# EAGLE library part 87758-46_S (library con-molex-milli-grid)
HEADER
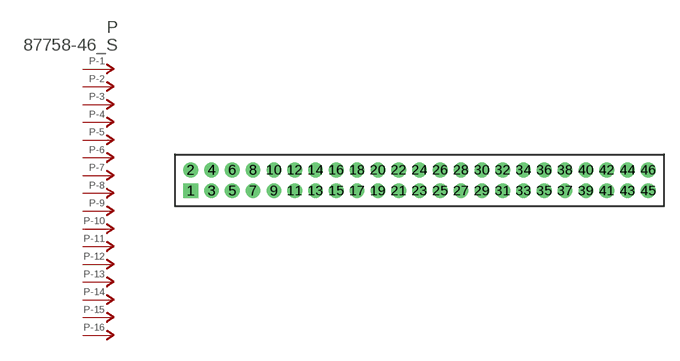
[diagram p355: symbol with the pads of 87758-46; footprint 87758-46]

Designator prefix P; gates -1=P-NV -2=P-N -3=P-N -4=P-N -5=P-N -6=P-N -7=P-N -8=P-N -9=P-N -10=P-N -11=P-N -12=P-N -13=P-N -14=P-N -15=P-N -16=P-N -17=P-N -18=P-N -19=P-N -20=P-N -21=P-N -22=P-N -23=P-N -24=P-N -25=P-N -26=P-N -27=P-N -28=P-N -29=P-N -30=P-N -31=P-N -32=P-N -33=P-N -34=P-N -35=P-N -36=P-N -37=P-N -38=P-N -39=P-N -40=P-N -41=P-N -42=P-N -43=P-N -44=P-N -45=P-N -46=P-N

## 87758-46_S  [87758-46]
1  -1:P  pas
2  -2:P  pas
3  -3:P  pas
4  -4:P  pas
5  -5:P  pas
6  -6:P  pas
7  -7:P  pas
8  -8:P  pas
9  -9:P  pas
10  -10:P  pas
11  -11:P  pas
12  -12:P  pas
13  -13:P  pas
14  -14:P  pas
15  -15:P  pas
16  -16:P  pas
17  -17:P  pas
18  -18:P  pas
19  -19:P  pas
20  -20:P  pas
21  -21:P  pas
22  -22:P  pas
23  -23:P  pas
24  -24:P  pas
25  -25:P  pas
26  -26:P  pas
27  -27:P  pas
28  -28:P  pas
29  -29:P  pas
30  -30:P  pas
31  -31:P  pas
32  -32:P  pas
33  -33:P  pas
34  -34:P  pas
35  -35:P  pas
36  -36:P  pas
37  -37:P  pas
38  -38:P  pas
39  -39:P  pas
40  -40:P  pas
41  -41:P  pas
42  -42:P  pas
43  -43:P  pas
44  -44:P  pas
45  -45:P  pas
46  -46:P  pas

## Footprint 87758-46 (pad centres in mm)
HEADER Dual Row, Vertical
drill 0.914 square: 1 -22,-1
drill 0.914: 2 -22,1; 3 -20,-1; 4 -20,1; 5 -18,-1; 6 -18,1; 7 -16,-1; 8 -16,1; 9 -14,-1; 10 -14,1; 11 -12,-1; 12 -12,1; 13 -10,-1; 14 -10,1; 15 -8,-1; 16 -8,1; 17 -6,-1; 18 -6,1; 19 -4,-1; 20 -4,1; 21 -2,-1; 22 -2,1; 23 0,-1; 24 0,1; 25 2,-1; 26 2,1; 27 4,-1; 28 4,1; 29 6,-1; 30 6,1; 31 8,-1; 32 8,1; 33 10,-1; 34 10,1; 35 12,-1; 36 12,1; 37 14,-1; 38 14,1; 39 16,-1; 40 16,1; 41 18,-1; 42 18,1; 43 20,-1; 44 20,1; 45 22,-1; 46 22,1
